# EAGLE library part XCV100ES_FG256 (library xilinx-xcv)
xcv100es_fg256 edit this description Auto generated by make-symbol-device-package-bsdl.ulp Rev. 26 Source: xcv100es_fg256.bsd
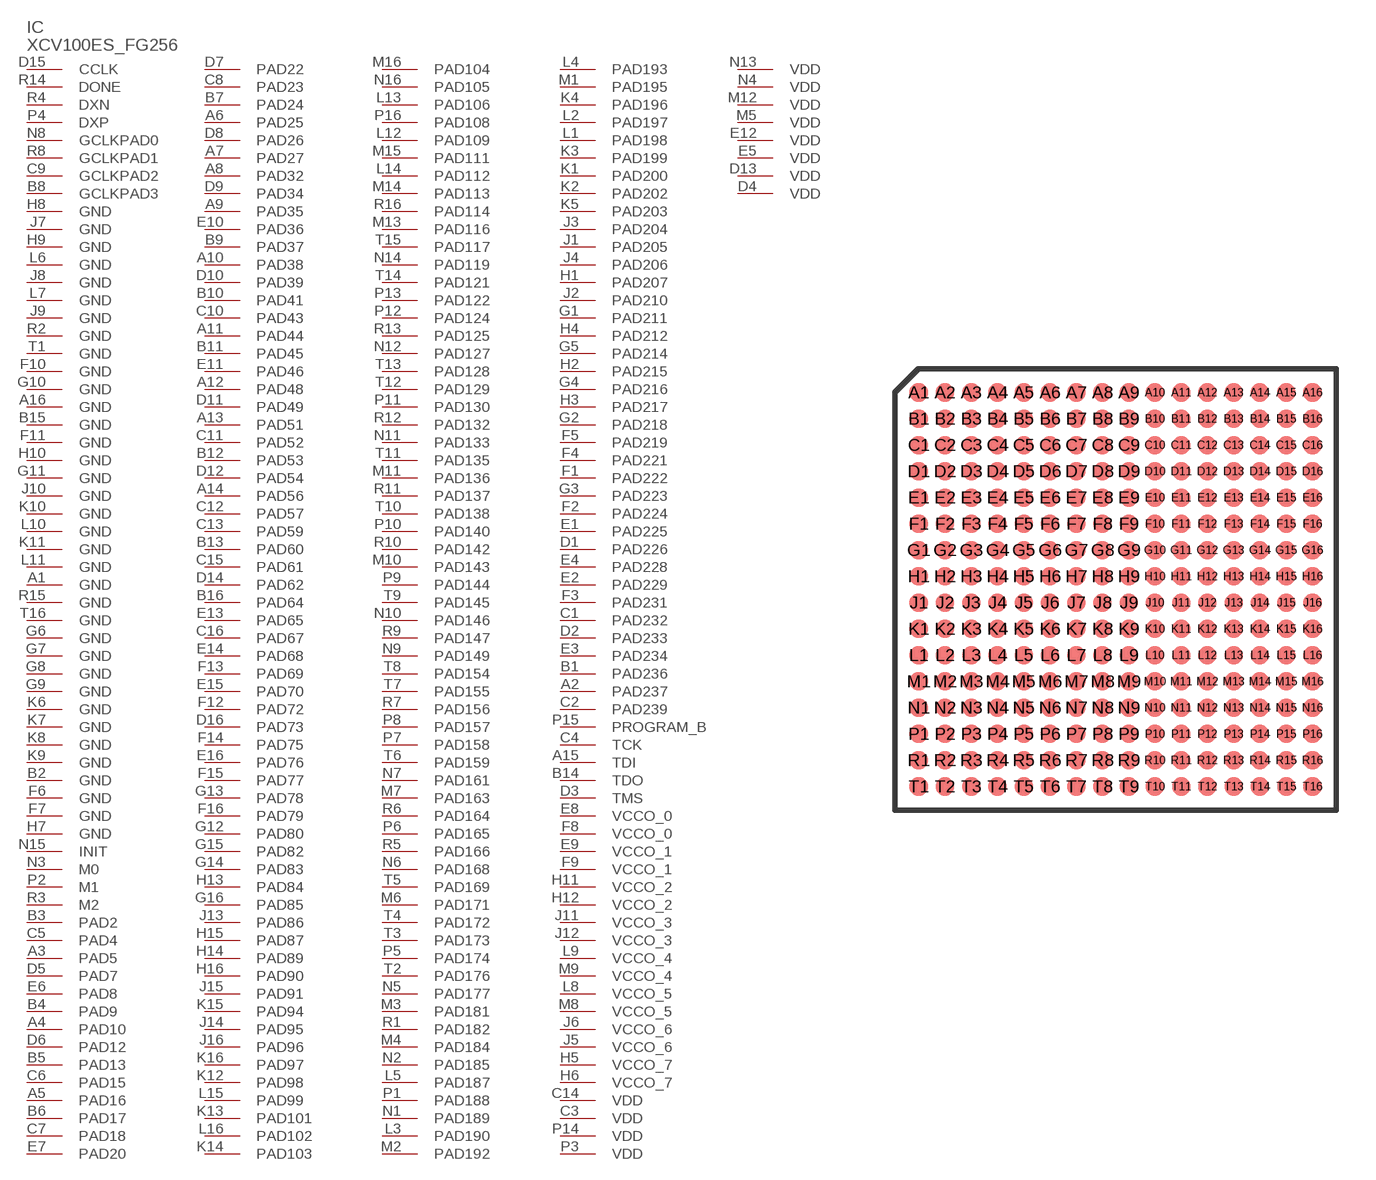
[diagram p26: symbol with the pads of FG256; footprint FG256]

Designator prefix IC

## XCV100ES_FG256 (OC_FARNELL: unknown; OC_NEWARK: unknown)  [FG256]
A1  GND  pwr
A2  PAD237
A3  PAD5
A4  PAD10
A5  PAD16
A6  PAD25
A7  PAD27
A8  PAD32
A9  PAD35
A10  PAD38
A11  PAD44
A12  PAD48
A13  PAD51
A14  PAD56
A15  TDI  in
A16  GND  pwr
B1  PAD236
B2  GND  pwr
B3  PAD2
B4  PAD9
B5  PAD13
B6  PAD17
B7  PAD24
B8  GCLKPAD3  in
B9  PAD37
B10  PAD41
B11  PAD45
B12  PAD53
B13  PAD60
B14  TDO  out
B15  GND  pwr
B16  PAD64
C1  PAD232
C2  PAD239
C3  VDD  pwr
C4  TCK  in
C5  PAD4
C6  PAD15
C7  PAD18
C8  PAD23
C9  GCLKPAD2  in
C10  PAD43
C11  PAD52
C12  PAD57
C13  PAD59
C14  VDD  pwr
C15  PAD61
C16  PAD67
D1  PAD226
D2  PAD233
D3  TMS  in
D4  VDD  pwr
D5  PAD7
D6  PAD12
D7  PAD22
D8  PAD26
D9  PAD34
D10  PAD39
D11  PAD49
D12  PAD54
D13  VDD  pwr
D14  PAD62
D15  CCLK
D16  PAD73
E1  PAD225
E2  PAD229
E3  PAD234
E4  PAD228
E5  VDD  pwr
E6  PAD8
E7  PAD20
E8  VCCO_0  pwr
E9  VCCO_1  pwr
E10  PAD36
E11  PAD46
E12  VDD  pwr
E13  PAD65
E14  PAD68
E15  PAD70
E16  PAD76
F1  PAD222
F2  PAD224
F3  PAD231
F4  PAD221
F5  PAD219
F6  GND  pwr
F7  GND  pwr
F8  VCCO_0  pwr
F9  VCCO_1  pwr
F10  GND  pwr
F11  GND  pwr
F12  PAD72
F13  PAD69
F14  PAD75
F15  PAD77
F16  PAD79
G1  PAD211
G2  PAD218
G3  PAD223
G4  PAD216
G5  PAD214
G6  GND  pwr
G7  GND  pwr
G8  GND  pwr
G9  GND  pwr
G10  GND  pwr
G11  GND  pwr
G12  PAD80
G13  PAD78
G14  PAD83
G15  PAD82
G16  PAD85
H1  PAD207
H2  PAD215
H3  PAD217
H4  PAD212
H5  VCCO_7  pwr
H6  VCCO_7  pwr
H7  GND  pwr
H8  GND  pwr
H9  GND  pwr
H10  GND  pwr
H11  VCCO_2  pwr
H12  VCCO_2  pwr
H13  PAD84
H14  PAD89
H15  PAD87
H16  PAD90
J1  PAD205
J2  PAD210
J3  PAD204
J4  PAD206
J5  VCCO_6  pwr
J6  VCCO_6  pwr
J7  GND  pwr
J8  GND  pwr
J9  GND  pwr
J10  GND  pwr
J11  VCCO_3  pwr
J12  VCCO_3  pwr
J13  PAD86
J14  PAD95
J15  PAD91
J16  PAD96
K1  PAD200
K2  PAD202
K3  PAD199
K4  PAD196
K5  PAD203
K6  GND  pwr
K7  GND  pwr
K8  GND  pwr
K9  GND  pwr
K10  GND  pwr
K11  GND  pwr
K12  PAD98
K13  PAD101
K14  PAD103
K15  PAD94
K16  PAD97
L1  PAD198
L2  PAD197
L3  PAD190
L4  PAD193
L5  PAD187
L6  GND  pwr
L7  GND  pwr
L8  VCCO_5  pwr
L9  VCCO_4  pwr
L10  GND  pwr
L11  GND  pwr
L12  PAD109
L13  PAD106
L14  PAD112
L15  PAD99
L16  PAD102
M1  PAD195
M2  PAD192
M3  PAD181
M4  PAD184
M5  VDD  pwr
M6  PAD171
M7  PAD163
M8  VCCO_5  pwr
M9  VCCO_4  pwr
M10  PAD143
M11  PAD136
M12  VDD  pwr
M13  PAD116
M14  PAD113
M15  PAD111
M16  PAD104
N1  PAD189
N2  PAD185
N3  M0  in
N4  VDD  pwr
N5  PAD177
N6  PAD168
N7  PAD161
N8  GCLKPAD0  in
N9  PAD149
N10  PAD146
N11  PAD133
N12  PAD127
N13  VDD  pwr
N14  PAD119
N15  INIT
N16  PAD105
P1  PAD188
P2  M1  in
P3  VDD  pwr
P4  DXP  pas
P5  PAD174
P6  PAD165
P7  PAD158
P8  PAD157
P9  PAD144
P10  PAD140
P11  PAD130
P12  PAD124
P13  PAD122
P14  VDD  pwr
P15  PROGRAM_B  in
P16  PAD108
R1  PAD182
R2  GND  pwr
R3  M2  in
R4  DXN  pas
R5  PAD166
R6  PAD164
R7  PAD156
R8  GCLKPAD1  in
R9  PAD147
R10  PAD142
R11  PAD137
R12  PAD132
R13  PAD125
R14  DONE
R15  GND  pwr
R16  PAD114
T1  GND  pwr
T2  PAD176
T3  PAD173
T4  PAD172
T5  PAD169
T6  PAD159
T7  PAD155
T8  PAD154
T9  PAD145
T10  PAD138
T11  PAD135
T12  PAD129
T13  PAD128
T14  PAD121
T15  PAD117
T16  GND  pwr

## Footprint FG256 (pad centres in mm)
Fine Pitch BGA (FG256) Auto generated by make-symbol-device-package-bsdl.ulp Rev. 26 Source: xcv100_fg256.bsd; fg256.pdf
smd 0.7 x 0.7: A1 -7.5,7.5; A2 -6.5,7.5; A3 -5.5,7.5; A4 -4.5,7.5; A5 -3.5,7.5; A6 -2.5,7.5; A7 -1.5,7.5; A8 -0.5,7.5; A9 0.5,7.5; A10 1.5,7.5; A11 2.5,7.5; A12 3.5,7.5; A13 4.5,7.5; A14 5.5,7.5; A15 6.5,7.5; A16 7.5,7.5; B1 -7.5,6.5; B2 -6.5,6.5; B3 -5.5,6.5; B4 -4.5,6.5; B5 -3.5,6.5; B6 -2.5,6.5; B7 -1.5,6.5; B8 -0.5,6.5; B9 0.5,6.5; B10 1.5,6.5; B11 2.5,6.5; B12 3.5,6.5; B13 4.5,6.5; B14 5.5,6.5; B15 6.5,6.5; B16 7.5,6.5; C1 -7.5,5.5; C2 -6.5,5.5; C3 -5.5,5.5; C4 -4.5,5.5; C5 -3.5,5.5; C6 -2.5,5.5; C7 -1.5,5.5; C8 -0.5,5.5; C9 0.5,5.5; C10 1.5,5.5; C11 2.5,5.5; C12 3.5,5.5; C13 4.5,5.5; C14 5.5,5.5; C15 6.5,5.5; C16 7.5,5.5; D1 -7.5,4.5; D2 -6.5,4.5; D3 -5.5,4.5; D4 -4.5,4.5; D5 -3.5,4.5; D6 -2.5,4.5; D7 -1.5,4.5; D8 -0.5,4.5; D9 0.5,4.5; D10 1.5,4.5; D11 2.5,4.5; D12 3.5,4.5; D13 4.5,4.5; D14 5.5,4.5; D15 6.5,4.5; D16 7.5,4.5; E1 -7.5,3.5; E2 -6.5,3.5; E3 -5.5,3.5; E4 -4.5,3.5; E5 -3.5,3.5; E6 -2.5,3.5; E7 -1.5,3.5; E8 -0.5,3.5; E9 0.5,3.5; E10 1.5,3.5; E11 2.5,3.5; E12 3.5,3.5; E13 4.5,3.5; E14 5.5,3.5; E15 6.5,3.5; E16 7.5,3.5; F1 -7.5,2.5; F2 -6.5,2.5; F3 -5.5,2.5; F4 -4.5,2.5; F5 -3.5,2.5; F6 -2.5,2.5; F7 -1.5,2.5; F8 -0.5,2.5; F9 0.5,2.5; F10 1.5,2.5; F11 2.5,2.5; F12 3.5,2.5; F13 4.5,2.5; F14 5.5,2.5; F15 6.5,2.5; F16 7.5,2.5; G1 -7.5,1.5; G2 -6.5,1.5; G3 -5.5,1.5; G4 -4.5,1.5; G5 -3.5,1.5; G6 -2.5,1.5; G7 -1.5,1.5; G8 -0.5,1.5; G9 0.5,1.5; G10 1.5,1.5; G11 2.5,1.5; G12 3.5,1.5; G13 4.5,1.5; G14 5.5,1.5; G15 6.5,1.5; G16 7.5,1.5; H1 -7.5,0.5; H2 -6.5,0.5; H3 -5.5,0.5; H4 -4.5,0.5; H5 -3.5,0.5; H6 -2.5,0.5; H7 -1.5,0.5; H8 -0.5,0.5; H9 0.5,0.5; H10 1.5,0.5; H11 2.5,0.5; H12 3.5,0.5; H13 4.5,0.5; H14 5.5,0.5; H15 6.5,0.5; H16 7.5,0.5; J1 -7.5,-0.5; J2 -6.5,-0.5; J3 -5.5,-0.5; J4 -4.5,-0.5; J5 -3.5,-0.5; J6 -2.5,-0.5; J7 -1.5,-0.5; J8 -0.5,-0.5; J9 0.5,-0.5; J10 1.5,-0.5; J11 2.5,-0.5; J12 3.5,-0.5; J13 4.5,-0.5; J14 5.5,-0.5; J15 6.5,-0.5; J16 7.5,-0.5; K1 -7.5,-1.5; K2 -6.5,-1.5; K3 -5.5,-1.5; K4 -4.5,-1.5; K5 -3.5,-1.5; K6 -2.5,-1.5; K7 -1.5,-1.5; K8 -0.5,-1.5; K9 0.5,-1.5; K10 1.5,-1.5; K11 2.5,-1.5; K12 3.5,-1.5; K13 4.5,-1.5; K14 5.5,-1.5; K15 6.5,-1.5; K16 7.5,-1.5; L1 -7.5,-2.5; L2 -6.5,-2.5; L3 -5.5,-2.5; L4 -4.5,-2.5; L5 -3.5,-2.5; L6 -2.5,-2.5; L7 -1.5,-2.5; L8 -0.5,-2.5; L9 0.5,-2.5; L10 1.5,-2.5; L11 2.5,-2.5; L12 3.5,-2.5; L13 4.5,-2.5; L14 5.5,-2.5; L15 6.5,-2.5; L16 7.5,-2.5; M1 -7.5,-3.5; M2 -6.5,-3.5; M3 -5.5,-3.5; M4 -4.5,-3.5; M5 -3.5,-3.5; M6 -2.5,-3.5; M7 -1.5,-3.5; M8 -0.5,-3.5; M9 0.5,-3.5; M10 1.5,-3.5; M11 2.5,-3.5; M12 3.5,-3.5; M13 4.5,-3.5; M14 5.5,-3.5; M15 6.5,-3.5; M16 7.5,-3.5; N1 -7.5,-4.5; N2 -6.5,-4.5; N3 -5.5,-4.5; N4 -4.5,-4.5; N5 -3.5,-4.5; N6 -2.5,-4.5; N7 -1.5,-4.5; N8 -0.5,-4.5; N9 0.5,-4.5; N10 1.5,-4.5; N11 2.5,-4.5; N12 3.5,-4.5; N13 4.5,-4.5; N14 5.5,-4.5; N15 6.5,-4.5; N16 7.5,-4.5; P1 -7.5,-5.5; P2 -6.5,-5.5; P3 -5.5,-5.5; P4 -4.5,-5.5; P5 -3.5,-5.5; P6 -2.5,-5.5; P7 -1.5,-5.5; P8 -0.5,-5.5; P9 0.5,-5.5; P10 1.5,-5.5; P11 2.5,-5.5; P12 3.5,-5.5; P13 4.5,-5.5; P14 5.5,-5.5; P15 6.5,-5.5; P16 7.5,-5.5; R1 -7.5,-6.5; R2 -6.5,-6.5; R3 -5.5,-6.5; R4 -4.5,-6.5; R5 -3.5,-6.5; R6 -2.5,-6.5; R7 -1.5,-6.5; R8 -0.5,-6.5; R9 0.5,-6.5; R10 1.5,-6.5; R11 2.5,-6.5; R12 3.5,-6.5; R13 4.5,-6.5; R14 5.5,-6.5; R15 6.5,-6.5; R16 7.5,-6.5; T1 -7.5,-7.5; T2 -6.5,-7.5; T3 -5.5,-7.5; T4 -4.5,-7.5; T5 -3.5,-7.5; T6 -2.5,-7.5; T7 -1.5,-7.5; T8 -0.5,-7.5; T9 0.5,-7.5; T10 1.5,-7.5; T11 2.5,-7.5; T12 3.5,-7.5; T13 4.5,-7.5; T14 5.5,-7.5; T15 6.5,-7.5; T16 7.5,-7.5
